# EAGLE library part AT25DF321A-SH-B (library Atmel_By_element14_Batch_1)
SPI Serial EEPROMs
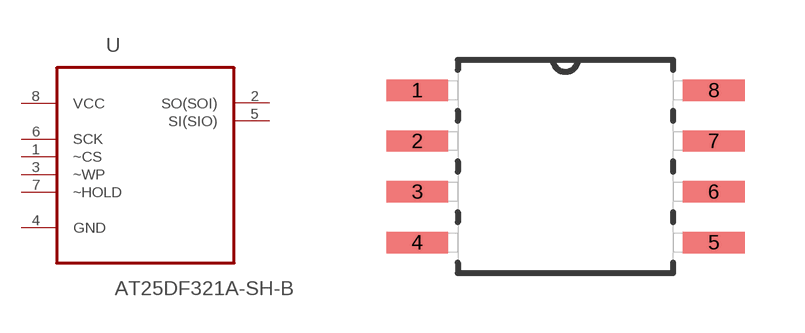
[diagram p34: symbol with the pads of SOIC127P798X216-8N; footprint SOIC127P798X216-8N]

Designator prefix U

## AT25DF321A-SH-B (MPN: AT25DF321A-SH-B; OC_FARNELL: 1841583; OC_NEWARK: 12T1349; PACKAGE: SOIC-8; SUPPLIER: Atmel)  [SOIC127P798X216-8N]
1  ~CS  in
2  SO(SOI)
3  ~WP  in
4  GND  pas
5  SI(SIO)
6  SCK  in
7  ~HOLD  in
8  VCC  pwr

## Footprint SOIC127P798X216-8N (pad centres in mm)
smd 1.549 x 0.533: 1 -3.708,1.905; 2 -3.708,0.635; 3 -3.708,-0.635; 4 -3.708,-1.905; 5 3.708,-1.905; 6 3.708,-0.635; 7 3.708,0.635; 8 3.708,1.905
